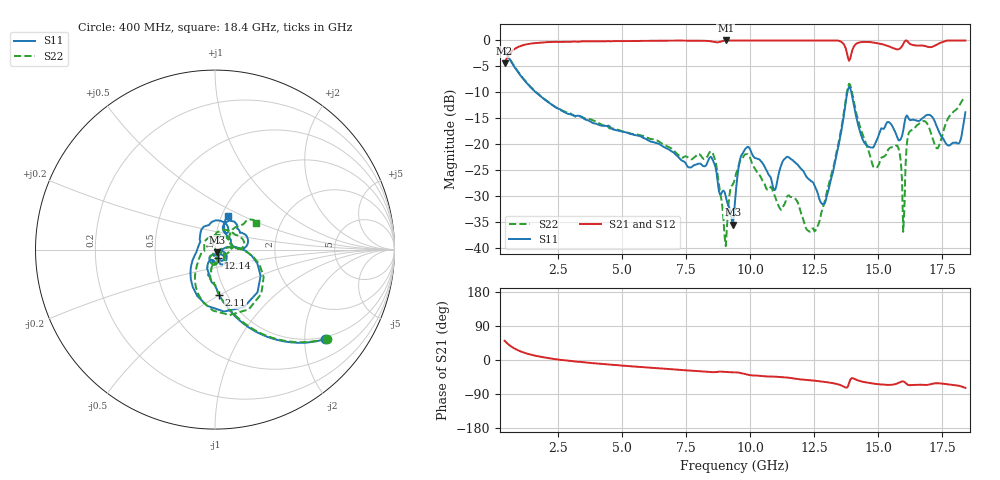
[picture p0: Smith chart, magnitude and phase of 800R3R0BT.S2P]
!  American Technical Ceramics  Date:  10/25/10
!  One Norden Lane
!  Huntington Station,  NY.  11746-2102
!  Tel:  (631) 622-4700  Fax:  (631) 622-4748
!  Part Number  800R3R0BT  Mounting Orientation: Vertical
!  Description: Ultra Low ESR Microwave Capacitor
!  Application: Coupling, Bypass, Tuning, DC Block, Filters, Matching
# GHZ S DB R 50
! Freq  |S11|  S11 Ph  |S21|  S21 Ph  |S12|  S12 Ph  |S22|  S22 Ph
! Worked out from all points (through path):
!   401 points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, 400 MHz to 18.4 GHz, reference 50 ohm
!   highest |S21| = 0.00 dB at 9.04 GHz (marker M1); lowest = -4.4 dB at 400 MHz (marker M2)
!   group delay of S21, straight-line fit = 14.2 ps
!   lowest |S11| = -35.5 dB at 9.31 GHz (marker M3), VSWR 1.03, Z = 51.1 - j1.31 ohm
!   |S11| at or under -10 dB: 1.621 GHz to 13.79 GHz (12.17 GHz wide, 158 % of centre); 13.95 GHz to end of sweep
!   |S22| runs from -39.6 to -2.0 dB; largest |S21 - S12| = 0.0036
!   S11 on the Smith chart (normalised r, x): 400 MHz: 0.94, -2.49; 2.11 GHz: 0.92, -0.50; 12.14 GHz: 1.03, -0.10; 18.4 GHz: 1.08, +0.42
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0.4  -2.05 -39.3  -4.40 50.6  -4.41 50.6  -1.97 -38.5
2.11  -11.90 -84.7  -0.32 4.9  -0.33 5.0  -11.85 -84.8
3.415  -14.78 -95.8  -0.18 -5.4  -0.19 -5.5  -14.74 -94.0
6.43  -19.92 -114.8  -0.06 -21.9  -0.06 -21.8  -19.48 -101.1
8.5  -22.70 -109.7  -0.20 -32.1  -0.19 -32.1  -21.51 -98.2
9.04  -30.05 -99.6  0.00 -31.2  -0.01 -31.2  -39.64 -55.4
9.31  -35.48 -49.8  -0.01 -32.5  -0.01 -32.5  -27.80 -29.3
9.4  -31.02 -15.7  -0.01 -32.5  -0.01 -32.5  -26.44 -26.4
9.85  -20.68 -52.0  -0.01 -37.9  -0.01 -37.9  -21.91 -56.6
10.93  -28.84 -60.5  -0.01 -43.8  -0.01 -43.8  -29.69 -83.4
11.425  -22.42 -51.2  -0.01 -46.0  -0.01 -46.0  -30.15 -59.5
12.145  -25.87 -67.8  -0.01 -52.4  -0.01 -52.4  -35.87 -77.2
12.415  -27.20 -61.8  -0.01 -53.8  -0.01 -53.9  -36.25 -45.1
12.955  -30.62 -10.2  -0.01 -58.3  -0.01 -58.4  -29.89 5.8
13.855  -8.91 -63.3  -3.92 -61.5  -3.91 -61.6  -8.35 -60.5
14.575  -20.36 173.2  -0.29 -59.8  -0.28 -59.9  -20.63 -155.2
15.43  -15.80 76.0  -1.17 -65.8  -1.17 -65.9  -20.78 58.1
15.79  -19.25 57.2  -1.69 -60.3  -1.68 -60.5  -20.85 0.7
15.97  -17.38 71.1  -0.71 -56.4  -0.71 -56.5  -36.86 -50.6
16.24  -15.36 43.7  -0.67 -66.3  -0.66 -66.5  -17.48 48.3
17.32  -17.04 1.2  -0.70 -61.4  -0.69 -61.5  -20.78 26.6
18.4  -13.83 68.4  -0.01 -73.6  -0.01 -73.8  -11.30 32.9
